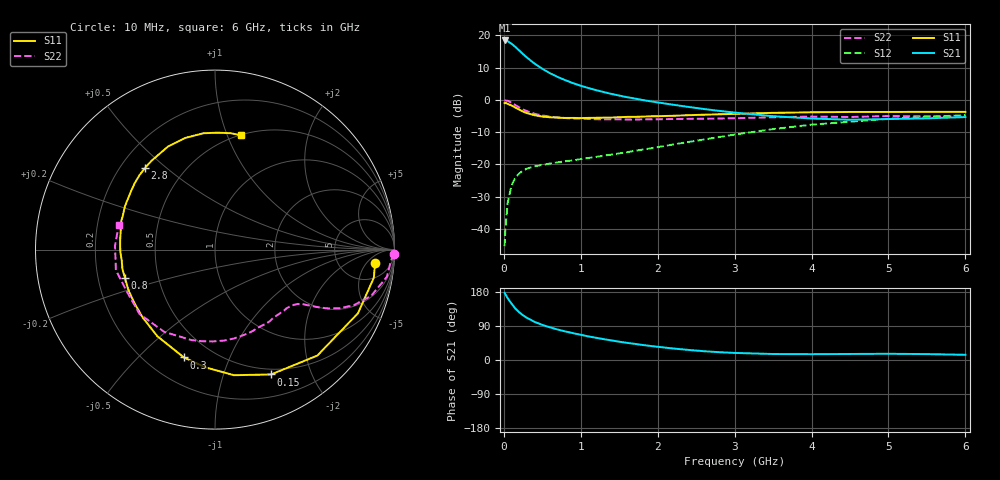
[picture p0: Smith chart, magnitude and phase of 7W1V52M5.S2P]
! Infineon Technologies  Discrete & RF Semiconductors
! BFS17W
! Si NPN RF Bipolar Junction Transistor in SOT323
! VCE = 1.5 V  IC = 2.5 mA
! Common Emitter S-Parameters:  August  1999
# GHz  S  MA  R  50
!  f  S11  S21  S12  S22
! GHz  MAG  ANG  MAG  ANG  MAG  ANG  MAG  ANG
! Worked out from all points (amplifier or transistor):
!   36 points, 10 MHz to 6 GHz, reference 50 ohm
!   highest |S21| = 18.5 dB at 10 MHz (marker M1)
!   |S21| within 3 dB of that: start of sweep to 194.8 MHz
!   unconditionally stable (mu >= 1): 720.9 MHz to end of sweep
!   at 250 MHz: K = 0.42, MSG = 18.1 dB, |S12| = -21.9 dB
!   at 1.4 GHz: K = 1.35, MAG = 5.9 dB, |S12| = -17.0 dB
!   at 6 GHz: K = 1.12, MAG = -2.4 dB, |S12| = -4.7 dB
!   S11 on the Smith chart (normalised r, x): 10 MHz: 11, -9; 150 MHz: 0.44, -1.45; 300 MHz: 0.35, -0.69; 800 MHz: 0.32, -0.14; 2.8 GHz: 0.30, +0.43; 6 GHz: 0.50, +1.12
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0.01  0.8944 -4.8  8.375 177.3  0.0054 85.3  0.9968 -1.3
0.02  0.8988 -10.0  8.335 173.4  0.0099 88.0  0.982 -3.7
0.05  0.872 -24.0  8.146 163.2  0.0255 78.8  0.9694 -9.0
0.1  0.8208 -46.0  7.445 148.6  0.0472 65.9  0.9076 -16.5
0.15  0.7626 -65.8  6.648 135.8  0.0629 56.5  0.8336 -21.8
0.2  0.7078 -81.4  5.85 125.9  0.0728 50.9  0.7679 -25.2
0.25  0.6582 -94.7  5.137 117.8  0.0802 45.8  0.7116 -27.4
0.3  0.6253 -106.1  4.55 111.2  0.0862 43.1  0.6714 -28.8
0.4  0.5797 -123.7  3.662 100.6  0.0934 39.6  0.6103 -30.7
0.5  0.5524 -137.0  3.047 92.7  0.0983 38.4  0.5753 -31.9
0.6  0.5386 -147.0  2.596 86.1  0.1032 38.5  0.5512 -33.3
0.8  0.5261 -162.4  2.024 75.3  0.112 40.1  0.5242 -37.2
0.9  0.527 -168.1  1.821 70.8  0.1153 41.6  0.5157 -39.2
1.1  0.5273 -178.5  1.53 62.2  0.1259 44.2  0.5074 -44.2
1.3  0.5318 173.1  1.325 54.9  0.1371 47.1  0.5 -49.9
1.6  0.5462 162.7  1.106 45.3  0.1547 50.5  0.4972 -58.7
2.2  0.5685 145.8  0.844 30.4  0.2036 55.9  0.5066 -78.1
2.8  0.5994 130.5  0.677 20.6  0.266 56.6  0.5159 -98.3
3.5  0.6312 114.5  0.56 15.8  0.3534 52.7  0.5387 -121.7
4.5  0.6515 95.6  0.493 15.9  0.4602 41.2  0.5442 -155.1
5.5  0.6544 82.3  0.519 15.6  0.5465 29.6  0.5575 177.8
6  0.6529 77.2  0.543 13.7  0.5808 24.0  0.5534 165.9
